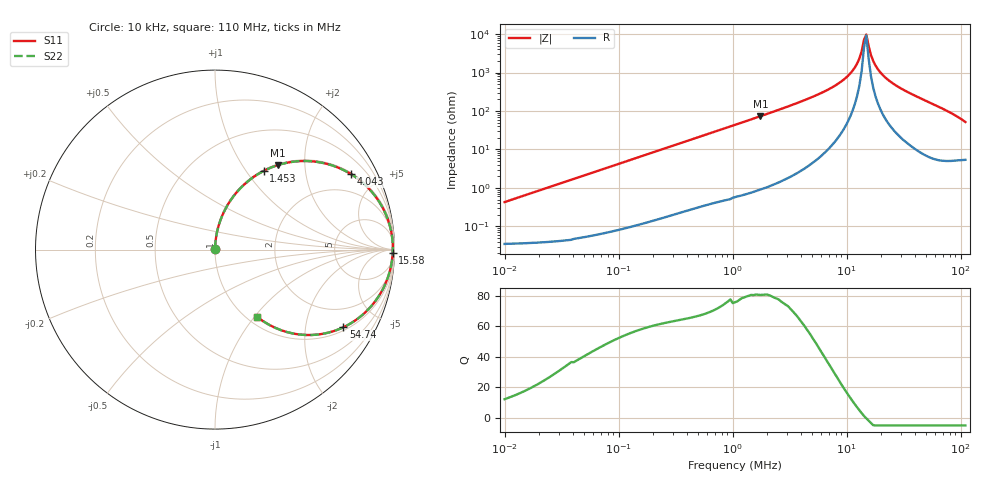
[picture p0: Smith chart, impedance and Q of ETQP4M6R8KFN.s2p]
! *** S-Parameter ***
!Copyright (C)  Panasonic Industry Corporation
!Power Inductors for Automotive application
!Parts No. ETQP4M6R8KFN
# HZ S RI R 50.000000
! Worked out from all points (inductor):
!   201 points, 10 kHz to 110 MHz, reference 50 ohm
!   read as one part in series: L = 6.8 uH near 10.48 kHz
!   highest Q = 80.6 at 1.75 MHz (marker M1), where L = 6.66 uH
!   self-resonance near 14.2 MHz
!   S11 on the Smith chart (normalised r, x): 10 kHz: 1.00, +0.01; 1.453 MHz: 1.02, +1.21; 4.043 MHz: 1.06, +3.60; 15.58 MHz: 48, -86; 54.74 MHz: 1.12, -3.22; 110 MHz: 1.11, -1.03
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10000  0.000368 0.00427  0.9996 -0.00427  0.9996 -0.00427  0.000368 0.00427
48644.84  0.000944 0.0206  0.9991 -0.0206  0.9991 -0.0206  0.000944 0.0206
225874.2  0.0104 0.0938  0.9896 -0.0938  0.9896 -0.0938  0.0104 0.0938
1048809  0.163 0.3628  0.837 -0.3628  0.837 -0.3628  0.163 0.3628
1452597  0.2708 0.4382  0.7292 -0.4382  0.7292 -0.4382  0.2708 0.4382
1749738  0.3506 0.471  0.6494 -0.471  0.6494 -0.471  0.3506 0.471
4042949  0.7602 0.419  0.2398 -0.419  0.2398 -0.419  0.7602 0.419
5101914  0.8455 0.3518  0.1545 -0.3518  0.1545 -0.3518  0.8455 0.3518
8124614  0.9518 0.1966  0.0482 -0.1966  0.0482 -0.1966  0.9518 0.1966
1.0741e7  0.9813 0.1028  0.0187 -0.1028  0.0187 -0.1028  0.9813 0.1028
1.293816e7  0.9898 0.0412  0.0102 -0.0412  0.0102 -0.0412  0.9898 0.0412
1.355437e7  0.9907 0.0258  0.0093 -0.0258  0.0093 -0.0258  0.9907 0.0258
1.419993e7  0.9909 0.0105  0.00913 -0.0105  0.00913 -0.0105  0.9909 0.0105
1.487624e7  0.9905 -0.00349  0.00949 0.00349  0.00949 0.00349  0.9905 -0.00349
1.558476e7  0.9901 -0.0175  0.00992 0.0175  0.00992 0.0175  0.9901 -0.0175
1.632703e7  0.9891 -0.0328  0.0109 0.0328  0.0109 0.0328  0.9891 -0.0328
1.79193e7  0.9857 -0.0633  0.0143 0.0633  0.0143 0.0633  0.9857 -0.0633
2.368988e7  0.9631 -0.1559  0.0369 0.1559  0.0369 0.1559  0.9631 -0.1559
3.437309e7  0.8952 -0.2842  0.1048 0.2842  0.1048 0.2842  0.8952 -0.2842
5.473791e7  0.7146 -0.4332  0.2854 0.4332  0.2854 0.4332  0.7146 -0.4332
7.942257e7  0.4706 -0.4731  0.5294 0.4731  0.5294 0.4731  0.4706 -0.4731
1.1e8  0.2342 -0.3745  0.7658 0.3745  0.7658 0.3745  0.2342 -0.3745
